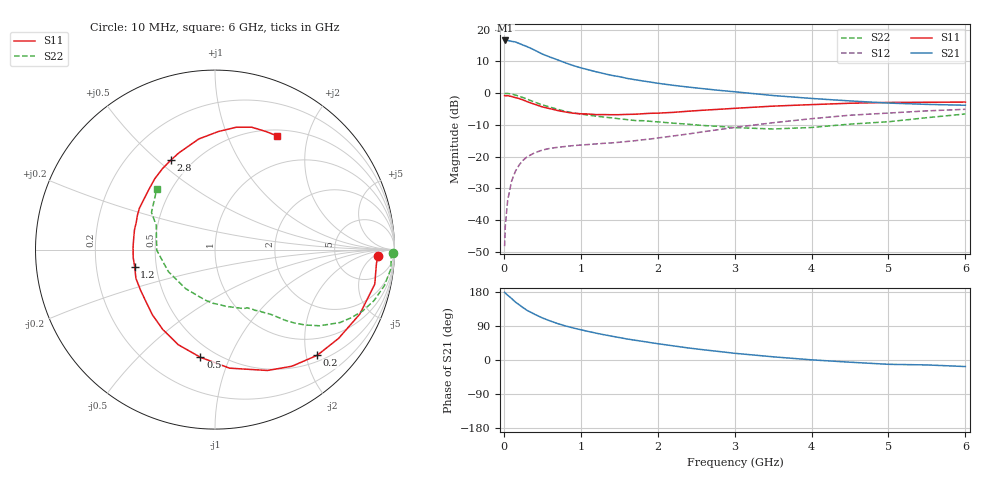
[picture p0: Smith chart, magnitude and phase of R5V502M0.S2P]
! SIEMENS Small Signal Semiconductors
! BFR183
! Si NPN RF Bipolar Junction Transistor in SOT23
! VCE = 0.5 V  IC = 2 mA
! Common Emitter S-Parameters:  May  1996
# GHz  S  MA  R  50
!  f  S11  S21  S12  S22
! GHz  MAG  ANG  MAG  ANG  MAG  ANG  MAG  ANG
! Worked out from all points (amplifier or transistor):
!   36 points, 10 MHz to 6 GHz, reference 50 ohm
!   highest |S21| = 16.6 dB at 20 MHz (marker M1)
!   |S21| within 3 dB of that: start of sweep to 396.9 MHz
!   unconditionally stable (mu >= 1): 1.317 GHz to 3.662 GHz
!   at 250 MHz: K = 0.24, MSG = 18.1 dB, |S12| = -21.2 dB
!   at 1.4 GHz: K = 1.04, MAG = 9.4 dB, |S12| = -15.7 dB
!   at 6 GHz: K = 0.99, MSG = 0.6 dB, |S12| = -5.1 dB
!   S11 on the Smith chart (normalised r, x): 10 MHz: 18, -8; 200 MHz: 0.62, -2.21; 500 MHz: 0.41, -0.78; 1.2 GHz: 0.38, -0.09; 2.8 GHz: 0.38, +0.55; 6 GHz: 0.58, +1.53
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0.01  0.911 -2.4  6.627 178.6  0.0039 89.7  0.993 -1.2
0.02  0.9028 -4.8  6.726 176.3  0.0084 89.2  0.9825 -2.4
0.05  0.9107 -12.2  6.725 171.0  0.0206 82.2  0.9858 -6.2
0.1  0.8829 -24.1  6.519 162.5  0.0409 76.6  0.965 -12.0
0.15  0.8478 -35.7  6.37 153.0  0.0588 69.7  0.9304 -17.8
0.2  0.8191 -46.0  6.024 145.6  0.0741 64.2  0.8915 -22.5
0.25  0.7784 -56.6  5.689 138.2  0.0875 59.1  0.8483 -26.6
0.3  0.7344 -66.5  5.394 131.2  0.0988 55.1  0.8059 -30.3
0.4  0.6655 -83.0  4.743 120.7  0.1149 48.0  0.7204 -36.1
0.5  0.6055 -97.7  4.112 111.1  0.1266 43.1  0.6531 -40.0
0.6  0.5682 -111.1  3.686 103.2  0.1351 39.5  0.6013 -42.8
0.7  0.5314 -123.3  3.327 96.1  0.1401 37.1  0.555 -45.2
0.8  0.5035 -133.9  2.991 90.0  0.1445 35.4  0.5167 -47.0
1.1  0.4689 -159.9  2.321 75.2  0.1552 33.6  0.4499 -51.6
1.2  0.4576 -168.1  2.161 70.8  0.1584 33.5  0.4332 -53.2
1.6  0.4619 166.2  1.705 55.5  0.173 36.4  0.382 -59.4
2.2  0.4968 138.3  1.325 37.4  0.2113 40.3  0.3363 -72.7
2.8  0.5559 116.2  1.103 22.4  0.2664 40.2  0.2988 -92.6
3.5  0.6232 98.3  0.915 8.4  0.3414 34.8  0.2722 -126.9
4.5  0.6917 80.2  0.752 -5.8  0.4482 22.7  0.3246 -179.4
5.5  0.7164 66.8  0.664 -13.0  0.5247 9.9  0.4099 149.7
6  0.7222 61.3  0.643 -17.3  0.5554 1.7  0.469 133.7
